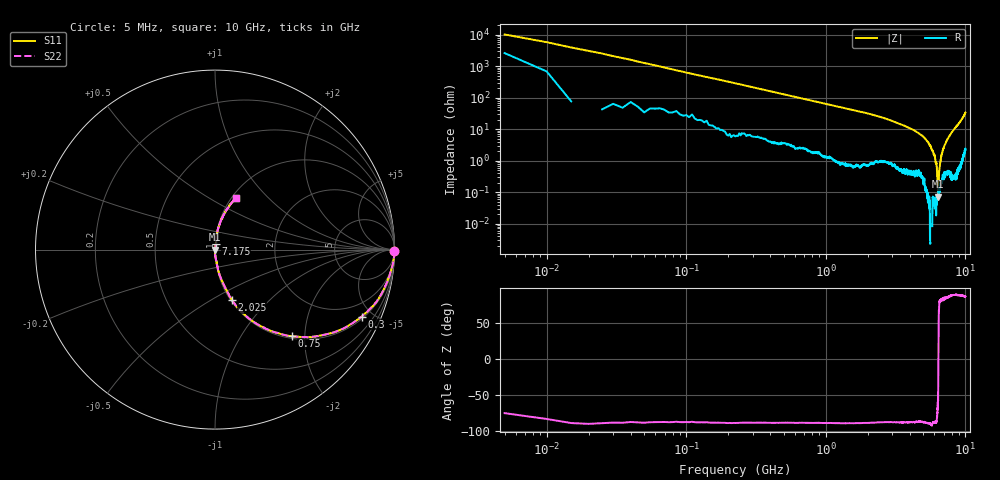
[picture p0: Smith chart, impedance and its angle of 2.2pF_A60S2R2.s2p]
! Amotech Co.,Ltd.
! http://www.amotech.co.kr/
! Part Number: A60S2R2
! These Parameters are Measured in Series Mode Connection
! Operation Temp=25[degC], DC Bias Voltage=0[V]
! Freq. Start=5[MHz] Stop=10[GHz], 2000[Steps]
! Date: Monday, July 13, 2020, 01:51:41
# GHZ S RI R 50.000000
!Freq.(Hz) S11(Real) S11(Imag) S21(Real) S21(Imag) S12(Real) S12(Imag) S22(Real) S22(Imag)
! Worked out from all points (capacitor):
!   2000 points, 5 MHz to 10 GHz, reference 50 ohm
!   read as one part in series: C = 2.49 pF near 55 MHz
!   lowest |Z| = 70.8 mohm at 6.395 GHz (marker M1)
!   series resonance near 6.406 GHz, so ESL is about 250 pH
!   S11 on the Smith chart (normalised r, x): 5 MHz: open; 300 MHz: 1.12, -4.32; 750 MHz: 1.04, -1.73; 2.025 GHz: 1.01, -0.62; 7.175 GHz: 1.01, +0.07; 10 GHz: 1.05, +0.67
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0.005  0.9975 -0.0093  0.00255 0.0093  0.00255 0.0093  0.9975 -0.0093
0.065  0.9855 -0.0986  0.0145 0.0986  0.0145 0.0986  0.9855 -0.0986
0.105  0.9677 -0.1579  0.0323 0.1579  0.0323 0.1579  0.9677 -0.1579
0.18  0.9231 -0.2535  0.0769 0.2535  0.0769 0.2535  0.9231 -0.2535
0.3  0.8173 -0.3731  0.1827 0.3731  0.1827 0.3731  0.8173 -0.3731
0.75  0.4287 -0.4834  0.5713 0.4834  0.5713 0.4834  0.4287 -0.4834
1.16  0.2398 -0.4181  0.7602 0.4181  0.7602 0.4181  0.2398 -0.4181
1.675  0.1323 -0.3296  0.8677 0.3296  0.8677 0.3296  0.1323 -0.3296
2.025  0.094 -0.2809  0.906 0.2809  0.906 0.2809  0.094 -0.2809
3.34  0.027 -0.1463  0.973 0.1463  0.973 0.1463  0.027 -0.1463
5.005  0.00516 -0.0565  0.9948 0.0565  0.9948 0.0565  0.00516 -0.0565
5.62  0.000721 -0.0298  0.9993 0.0298  0.9993 0.0298  0.000721 -0.0298
6.03  0.000689 -0.0146  0.9993 0.0146  0.9993 0.0146  0.000689 -0.0146
6.215  0.000441 -0.00743  0.9996 0.00743  0.9996 0.00743  0.000441 -0.00743
6.355  0.000627 -0.00122  0.9994 0.00122  0.9994 0.00122  0.000627 -0.00122
6.395  0.000644 -0.000293  0.9994 0.000293  0.9994 0.000293  0.000644 -0.000293
6.51  0.00114 0.00476  0.9989 -0.00476  0.9989 -0.00476  0.00114 0.00476
6.67  0.00206 0.0112  0.9979 -0.0112  0.9979 -0.0112  0.00206 0.0112
6.91  0.00382 0.0219  0.9962 -0.0219  0.9962 -0.0219  0.00382 0.0219
7.175  0.00446 0.0338  0.9955 -0.0338  0.9955 -0.0338  0.00446 0.0338
8.335  0.0132 0.1003  0.9868 -0.1003  0.9868 -0.1003  0.0132 0.1003
10  0.1181 0.2903  0.8819 -0.2903  0.8819 -0.2903  0.1181 0.2903
